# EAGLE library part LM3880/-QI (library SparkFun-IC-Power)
LM3880 Simple Power Sequencer Precision enable pin & 3 open-drain output flags Input Voltage Range of 2.7 V to 5.5 V Power-Up and Power-Down Control The timing sequence of the LM3880 is controlled entirely by the enable (EN) pin. Upon power up, all the flags are held low until this precision enable is pulled high LM3880MF-1XY (Timing Designator) AF: 16ms AE: 2ms AA: 10ms AB: 30ms AC: 60ms AD: 120ms SparkFun Products SparkFun 6 Degrees of Freedom Breakout - LSM303C (BOB-13303)
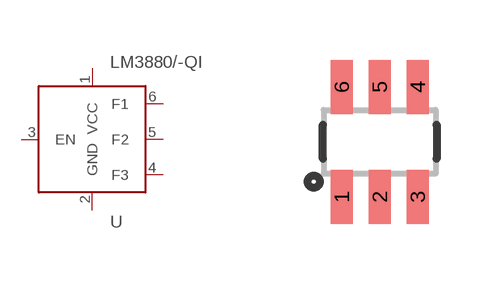
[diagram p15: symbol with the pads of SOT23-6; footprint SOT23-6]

Designator prefix U

## LM3880/-QI (PROD_ID: IC-12558; VALUE: LM3880)  [SOT23-6]
1  VCC
2  GND
3  EN
4  F3
5  F2
6  F1

## Footprint SOT23-6 (pad centres in mm)
smd 0.55 x 1.35: 1 -0.95,-1.375; 2 0,-1.375; 3 0.95,-1.375; 4 0.95,1.375; 5 0,1.375; 6 -0.95,1.375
